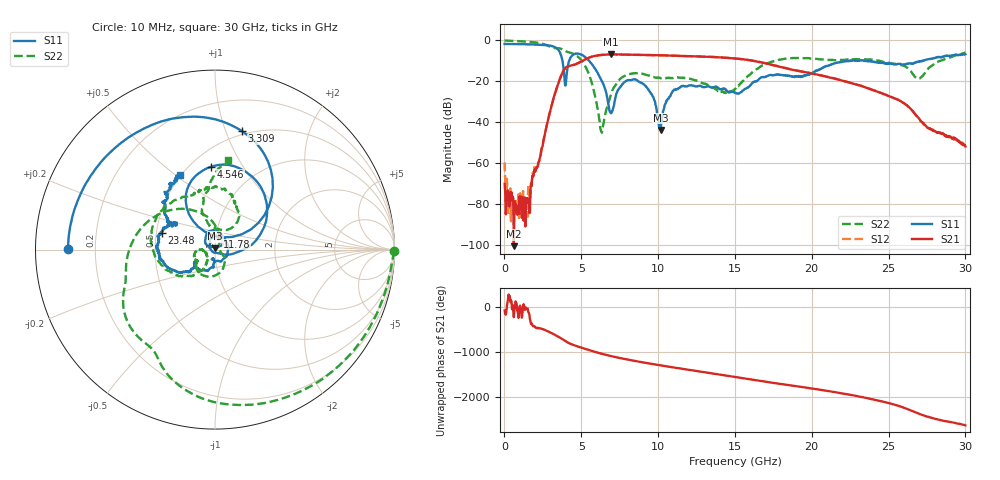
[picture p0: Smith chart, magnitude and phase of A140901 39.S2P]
!  2-Port S-parameters saved by WinCal
! VAR MeasName=S-Parameters (CALIBRATED_DATA) read from VNA (N5244A)
! VAR MeasDate=11/3/2014 9:33:38 AM
! VAR NAME=A140901 39
! VAR FILENAME=A140901 39.S2P
! VAR DATE=11/3/2014 9:33:38 AM
! VAR PHYS_PORTS=1,2
# Hz S RI R 50
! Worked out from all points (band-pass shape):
!   801 points, 10 MHz to 30 GHz, reference 50 ohm
!   highest |S21| = -6.83 dB at 6.908 GHz (marker M1); lowest = -100.6 dB at 609.8 MHz (marker M2)
!   |S21| within 3 dB of the highest: 5.11 GHz to 16.08 GHz (10.97 GHz wide, 104 % of centre)
!   lowest |S11| = -43.8 dB at 10.17 GHz (marker M3), VSWR 1.01, Z = 50.1 + j0.631 ohm
!   |S11| at or under -10 dB: 3.773 GHz to 4.209 GHz (436.8 MHz wide, 10.9 % of centre); 5.512 GHz to 22.38 GHz (16.87 GHz wide, 121 % of centre); 23.53 GHz to 27.23 GHz (3.706 GHz wide, 14.6 % of centre)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
!   |S22| runs from -45.1 to 0.0 dB; largest |S21 - S12| = 0.0027
!   S11 on the Smith chart (normalised r, x): 10 MHz: 0.10, +0.00; 3.309 GHz: 0.47, +1.14; 4.546 GHz: 0.63, +0.74; 11.78 GHz: 1.02, +0.15; 23.48 GHz: 0.53, +0.11; 30 GHz: 0.49, +0.52
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1e7  -0.8189 0.00272  4.69e-05 -0.000312  0.000511 0.000897  0.9962 -0.00852
6.098e8  -0.7911 0.197  -6.23e-06 7.01e-06  1.69e-05 -6.37e-05  0.8941 -0.3724
1.5095e9  -0.6529 0.4654  0.000115 -8.21e-05  -1.61e-06 4.96e-05  0.5213 -0.7677
3.3089e9  0.1515 0.6592  -0.0021 0.0535  -0.00221 0.0533  -0.3777 -0.5292
3.983675e9  -0.00996 0.0788  0.1494 -0.1538  0.1499 -0.1535  -0.5039 -0.2089
4.545988e9  -0.0196 0.4621  -0.1832 -0.176  -0.1825 -0.1761  -0.4542 0.0534
5.033325e9  0.2377 0.3737  -0.305 0.062  -0.3051 0.0613  -0.2265 0.2237
6.3079e9  0.1063 -0.021  0.3515 0.268  0.3506 0.2681  0.00547 0.00215
6.9077e9  -0.00432 -0.0166  0.4423 -0.1089  0.4419 -0.1084  0.0382 -0.023
8.519662e9  0.00989 0.1104  -0.2641 -0.3565  -0.2637 -0.3567  -0.0621 -0.1459
9.569312e9  0.0414 0.0262  -0.4309 0.074  -0.43 0.0727  -0.1049 -0.0825
1.001916e10  0.008 0.00651  -0.3548 0.251  -0.3543 0.2499  -0.1028 -0.069
1.016911e10  0.00141 0.00629  -0.3118 0.2992  -0.3116 0.2983  -0.0987 -0.0672
1.088138e10  -0.0284 0.0422  -0.0512 0.4205  -0.0516 0.4199  -0.1036 -0.0607
1.178108e10  0.014 0.0735  0.2705 0.3128  0.2709 0.3133  -0.1158 -0.0311
1.5005e10  -0.0118 -0.0504  -0.1855 -0.3097  -0.1856 -0.3096  -0.0416 -0.0497
1.729174e10  -0.0822 -0.1176  -0.1135 0.2331  -0.1149 0.2335  -0.2702 -0.1121
2.002832e10  -0.1215 -0.1004  0.1456 -0.0525  0.1468 -0.0525  -0.2426 0.2609
2.347718e10  -0.2978 0.0932  -0.0505 0.0504  -0.0507 0.0507  0.0163 0.3463
2.501416e10  -0.2226 0.1483  0.0423 0.0116  0.0423 0.0113  0.1122 0.2622
2.696351e10  -0.2677 0.1541  -0.00943 0.00814  -0.00954 0.00789  0.0174 0.1155
3e10  -0.1971 0.4157  -0.00142 -0.00213  -0.00124 -0.00223  0.0751 0.4978
